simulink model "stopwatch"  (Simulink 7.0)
settings: Solver=ode3  StartTime=0.0  StopTime=inf  FixedStep=1e-4  RelTol=1e-3
libraries: simulink x3

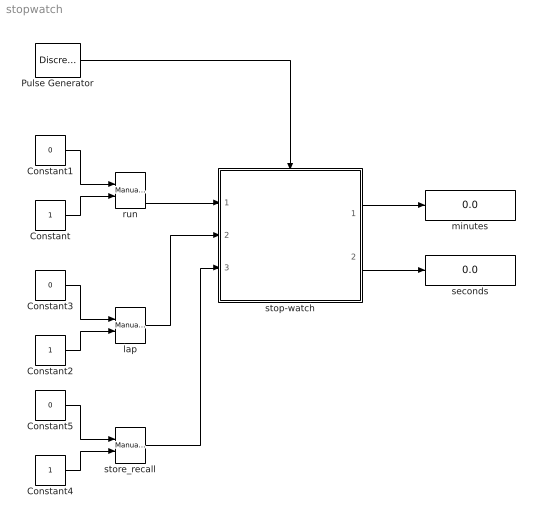
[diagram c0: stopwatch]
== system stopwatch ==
  Constant : Constant  OutDataType=sfix(16)  OutScaling=2^0
  Constant1 : Constant  Value=0  OutDataType=sfix(16)  OutScaling=2^0
  Constant2 : Constant  OutDataType=sfix(16)  OutScaling=2^0
  Constant3 : Constant  Value=0  OutDataType=sfix(16)  OutScaling=2^0
  Constant4 : Constant  OutDataType=sfix(16)  OutScaling=2^0
  Constant5 : Constant  Value=0  OutDataType=sfix(16)  OutScaling=2^0
  Pulse Generator : DiscretePulseGenerator  PulseType=Time based  Period=1  PulseWidth=50
  lap : simulink/Signal Routing/Manual Switch  SystemSampleTime=-1  sw=0  action=0  varsize=off
  minutes : Display
  run : simulink/Signal Routing/Manual Switch  SystemSampleTime=-1  sw=0  action=0  varsize=off
  seconds : Display
  stop-watch : Stateflow chart
  store_recall : simulink/Signal Routing/Manual Switch  SystemSampleTime=-1  sw=1  action=0  varsize=off
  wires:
  Constant1/1 -> run/1
  Constant/1 -> run/2
  stop-watch/1(minutes_out) -> minutes/1
  stop-watch/2(seconds_out) -> seconds/1
  run/1 -> stop-watch/1(run)
  Pulse Generator/1 -> stop-watch/Trigger
  Constant3/1 -> lap/1
  Constant2/1 -> lap/2
  lap/1 -> stop-watch/2(lap)
  Constant5/1 -> store_recall/1
  Constant4/1 -> store_recall/2
  store_recall/1 -> stop-watch/3(store_recall)

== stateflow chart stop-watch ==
  state Watch [parallel]
    state Stopped
    state Started
      state Count
      Count -> Count : tick[(seconds==59) & !lap]/ minutes:=minutes+1; seconds:=0;
      Count -> Count : tick[(seconds<59 & !lap)]/ seconds:=seconds+1;
      Count -> Count : tick[(seconds==59) & lap]/ minutes_out:=minutes+1; minutes:=minutes+1; seconds:=0; seconds_out:=0;
      Count -> Count : tick[(seconds<59 & lap)]/ seconds_out:=seconds+1; seconds:=seconds+1; minutes_out:=minutes;
      (default) -> Count
    (default) -> Stopped
    Stopped -> Started : [run]/ minutes:=0;minutes_out:=0; seconds:=0;seconds_out:=0;
    Started -> Stopped : [!run]
  state Memory [parallel]
    state Engaged
    state Disengaged
    Engaged -> Disengaged : [!store_recall]/ seconds:=mem_seconds; minutes:=mem_minutes; seconds_out:=mem_seconds; minutes_out:=mem_minutes;
    Disengaged -> Engaged : [store_recall]/ mem_seconds:=seconds; mem_minutes:=minutes;
    (junction 10) -> Engaged : [store_recall]
    (junction 10) -> Disengaged
    (default) -> (junction 10)
